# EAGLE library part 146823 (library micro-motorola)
MICROCONTROLLER/MEMORY DEVICE
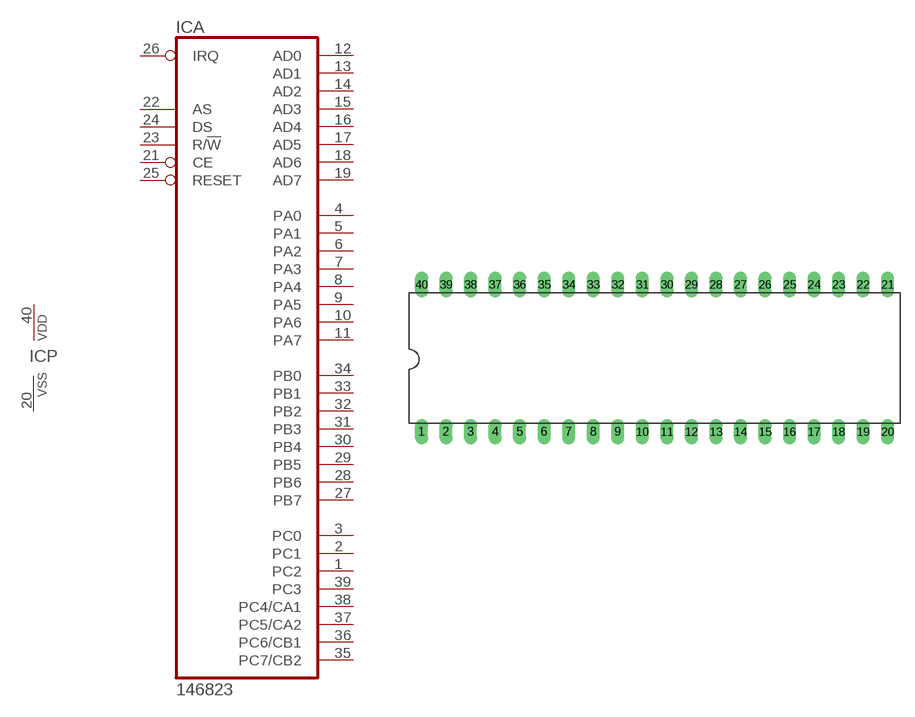
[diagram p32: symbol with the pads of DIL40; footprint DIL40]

Designator prefix IC; gates A=146823 P=VSSVDD

## 146823 (OC_FARNELL: unknown; OC_NEWARK: unknown)  [DIL40]
1  A:PC2
2  A:PC1
3  A:PC0
4  A:PA0
5  A:PA1
6  A:PA2
7  A:PA3
8  A:PA4
9  A:PA5
10  A:PA6
11  A:PA7
12  A:AD0
13  A:AD1
14  A:AD2
15  A:AD3
16  A:AD4
17  A:AD5
18  A:AD6
19  A:AD7
20  P:VSS  pwr
21  A:CE  in
22  A:AS  in
23  A:R/!W  in
24  A:DS  in
25  A:RESET  in
26  A:IRQ  out
27  A:PB7
28  A:PB6
29  A:PB5
30  A:PB4
31  A:PB3
32  A:PB2
33  A:PB1
34  A:PB0
35  A:PC7/CB2
36  A:PC6/CB1
37  A:PC5/CA2
38  A:PC4/CA1
39  A:PC3
40  P:VDD  pwr

## Footprint DIL40 (pad centres in mm)
Dual In Line Package
drill 0.813 long: 1 -24.13,-7.62; 2 -21.59,-7.62; 3 -19.05,-7.62; 4 -16.51,-7.62; 5 -13.97,-7.62; 6 -11.43,-7.62; 7 -8.89,-7.62; 8 -6.35,-7.62; 9 -3.81,-7.62; 10 -1.27,-7.62; 11 1.27,-7.62; 12 3.81,-7.62; 13 6.35,-7.62; 14 8.89,-7.62; 15 11.43,-7.62; 16 13.97,-7.62; 17 16.51,-7.62; 18 19.05,-7.62; 19 21.59,-7.62; 20 24.13,-7.62; 21 24.13,7.62; 22 21.59,7.62; 23 19.05,7.62; 24 16.51,7.62; 25 13.97,7.62; 26 11.43,7.62; 27 8.89,7.62; 28 6.35,7.62; 29 3.81,7.62; 30 1.27,7.62; 31 -1.27,7.62; 32 -3.81,7.62; 33 -6.35,7.62; 34 -8.89,7.62; 35 -11.43,7.62; 36 -13.97,7.62; 37 -16.51,7.62; 38 -19.05,7.62; 39 -21.59,7.62; 40 -24.13,7.62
